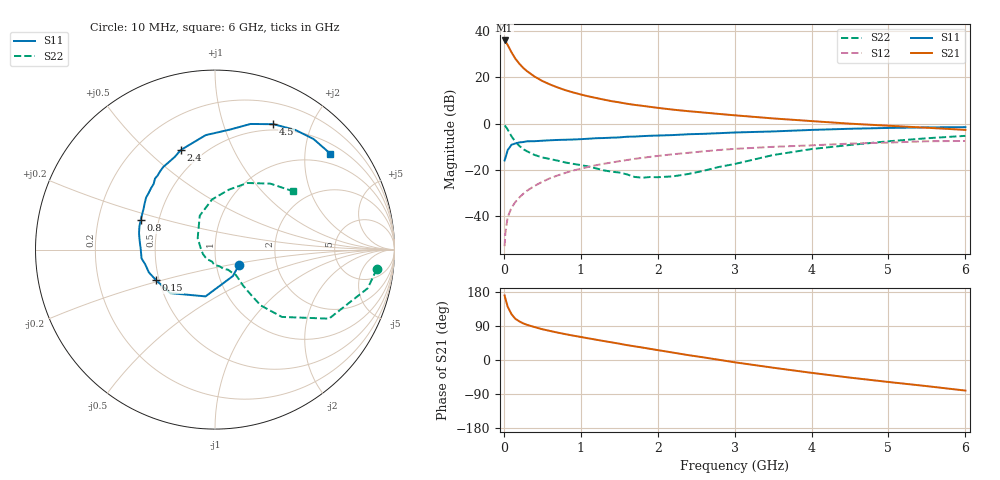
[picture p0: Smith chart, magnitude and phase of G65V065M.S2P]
! SIEMENS Small Signal Semiconductors
! BFG193
! Si NPN RF Bipolar Junction Transistor in SOT223
! VCE = 5 V  IC = 65 mA
! Common Emitter S-Parameters:  August  1996
# GHz  S  MA  R  50
!  f  S11  S21  S12  S22
! GHz  MAG  ANG  MAG  ANG  MAG  ANG  MAG  ANG
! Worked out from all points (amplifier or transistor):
!   36 points, 10 MHz to 6 GHz, reference 50 ohm
!   highest |S21| = 36.0 dB at 10 MHz (marker M1)
!   |S21| within 3 dB of that: start of sweep to 66.14 MHz
!   unconditionally stable (mu >= 1): 378.8 MHz to 2.356 GHz
!   at 250 MHz: K = 0.95, MSG = 27.4 dB, |S12| = -30.5 dB
!   at 1.4 GHz: K = 1.04, MAG = 12.0 dB, |S12| = -16.9 dB
!   at 6 GHz: K = 0.89, MSG = 2.4 dB, |S12| = -7.6 dB
!   S11 on the Smith chart (normalised r, x): 10 MHz: 1.29, -0.22; 150 MHz: 0.48, -0.19; 800 MHz: 0.40, +0.16; 2.4 GHz: 0.38, +0.64; 4.5 GHz: 0.43, +1.48; 6 GHz: 0.73, +2.59
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0.01  0.1589 -31.6  63.22 170.4  0.0022 83.6  0.9077 -6.9
0.02  0.1779 -56.1  60.82 162.2  0.0042 77.0  0.8778 -14.2
0.05  0.2659 -101.4  50.39 140.6  0.0094 73.0  0.7426 -31.2
0.1  0.3475 -135.7  34.89 120.7  0.0151 67.6  0.5287 -45.2
0.15  0.3698 -152.5  25.41 108.7  0.0199 68.3  0.4016 -50.7
0.2  0.3898 -161.0  19.93 102.1  0.0248 70.0  0.3307 -51.4
0.25  0.3976 -168.2  16.22 96.8  0.0298 69.8  0.2797 -51.8
0.3  0.4121 -173.1  13.71 92.9  0.0349 70.5  0.251 -52.0
0.4  0.4142 179.3  10.42 86.9  0.0446 71.0  0.2087 -51.1
0.5  0.4247 172.2  8.364 81.2  0.0547 69.7  0.1844 -50.6
0.6  0.4337 167.4  7.03 76.7  0.0652 68.7  0.1703 -51.6
0.7  0.4412 162.5  6.05 72.3  0.0751 67.3  0.157 -53.8
0.8  0.4457 158.1  5.289 68.2  0.0853 65.0  0.1433 -55.6
1.1  0.4689 146.7  3.884 57.1  0.1149 59.8  0.1171 -66.3
1.3  0.4855 139.7  3.302 50.0  0.1343 55.8  0.0967 -74.3
1.6  0.5179 130.2  2.689 39.3  0.162 48.9  0.0792 -95.9
2.2  0.5628 113.5  2 19.5  0.2162 35.3  0.0717 -160.2
2.4  0.5865 109.0  1.853 12.8  0.2323 31.0  0.0808 173.0
3.5  0.6743 82.8  1.291 -20.3  0.3129 3.9  0.2076 114.1
4.5  0.7708 65.0  0.994 -46.5  0.3675 -16.2  0.3431 76.9
5.5  0.8253 48.3  0.811 -69.0  0.4133 -39.6  0.4799 50.0
6  0.8359 39.7  0.729 -80.7  0.419 -53.1  0.5412 37.0
